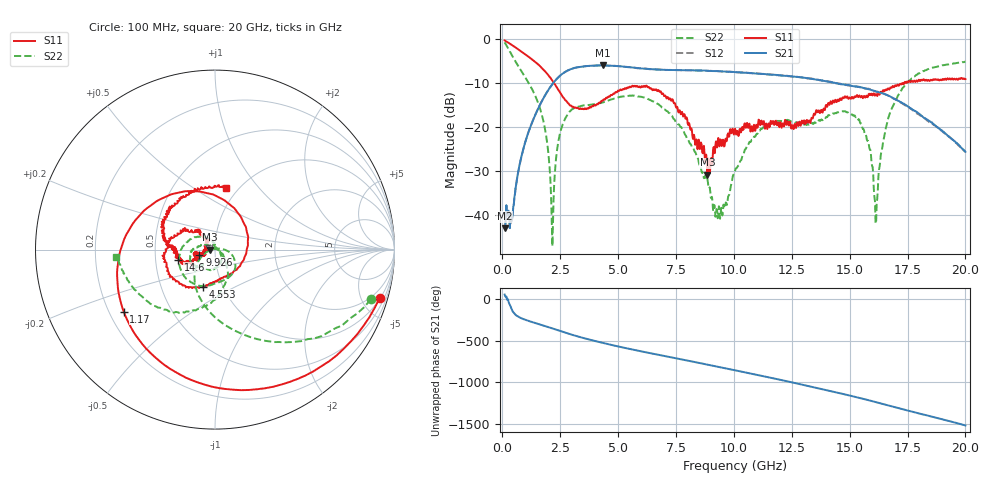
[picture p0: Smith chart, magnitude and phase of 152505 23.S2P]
!  2-Port S-parameters saved by WinCal
! VAR MeasName=S-Parameters (CALIBRATED_DATA) read from VNA (N5230C)
! VAR MeasDate=4/10/2015 9:30:38 AM
! VAR NAME=152505 23
! VAR FILENAME=152505 23.S2P
! VAR DATE=4/10/2015 9:30:38 AM
! VAR PHYS_PORTS=1,2
# Hz S DB R 50
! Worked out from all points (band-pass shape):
!   801 points, 100 MHz to 20 GHz, reference 50 ohm
!   highest |S21| = -6.03 dB at 4.329 GHz (marker M1); lowest = -42.9 dB at 100 MHz (marker M2)
!   |S21| within 3 dB of the highest: 2.363 GHz to 13.3 GHz (10.93 GHz wide, 140 % of centre)
!   lowest |S11| = -30.8 dB at 8.856 GHz (marker M3), VSWR 1.06, Z = 47.2 - j0.114 ohm
!   |S11| at or under -10 dB: 2.226 GHz to 17.36 GHz (15.13 GHz wide, 155 % of centre); 17.43299 GHz to 17.43998 GHz (6.986 MHz wide, 0.0401 % of centre)
!   |S22| runs from -47.0 to -0.8 dB; largest |S21 - S12| = 0.0065
!   S11 on the Smith chart (normalised r, x): 100 MHz: 1.08, -6.79; 1.17 GHz: 0.26, -0.29; 4.553 GHz: 0.81, -0.35; 9.926 GHz: 0.84, -0.05; 14.6 GHz: 0.66, -0.08; 20 GHz: 0.87, +0.69
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1e8  -0.39 -16.4  -42.90 55.0  -42.55 57.3  -0.80 -17.7
5.72625e8  -1.97 -79.4  -33.88 171.0  -33.87 171.4  -5.17 -64.8
1.169625e9  -4.22 -145.8  -20.56 94.2  -20.54 94.3  -10.31 -102.7
1.816375e9  -7.21 146.2  -13.09 38.3  -13.07 38.1  -19.67 -147.0
2.164625e9  -9.48 105.0  -10.26 7.1  -10.26 7.0  -46.95 93.7
2.562625e9  -12.70 51.2  -8.06 -29.5  -8.08 -29.6  -20.11 -16.9
3.43325e9  -15.92 -58.6  -6.32 -103.2  -6.31 -103.0  -15.20 -66.2
4.32875e9  -14.06 -100.2  -6.03 -166.3  -6.02 -166.3  -14.44 -90.8
4.552625e9  -13.30 -107.9  -6.06 178.8  -6.07 178.9  -14.02 -96.7
6.741625e9  -11.58 166.6  -6.99 49.8  -6.96 49.3  -14.78 174.9
8.856e9  -30.75 -177.6  -7.24 -68.8  -7.26 -68.7  -31.75 91.1
9.30375e9  -23.40 -167.2  -7.33 -94.0  -7.32 -94.2  -40.63 65.6
9.925625e9  -20.72 -160.7  -7.51 -129.8  -7.49 -129.9  -31.99 -19.0
1.005e10  -20.36 -156.9  -7.55 -137.1  -7.55 -137.2  -29.90 -23.1
1.19405e10  -19.67 -161.4  -8.26 112.0  -8.30 112.1  -18.59 -108.5
1.338325e10  -17.99 -152.1  -9.11 23.0  -9.06 23.1  -19.06 -129.8
1.460212e10  -13.49 -164.8  -10.28 -54.7  -10.18 -55.5  -16.47 -151.7
1.559712e10  -13.27 -179.8  -11.15 -121.7  -11.11 -121.5  -20.41 168.0
1.614438e10  -12.50 179.2  -11.95 -160.8  -11.98 -161.3  -41.67 26.0
1.669162e10  -11.45 173.8  -12.92 158.9  -12.99 157.5  -17.57 -57.9
1.805975e10  -9.52 138.5  -17.19 58.6  -17.41 59.4  -7.59 -122.8
2e10  -9.14 80.3  -25.60 -81.0  -25.65 -80.3  -5.19 -176.0
